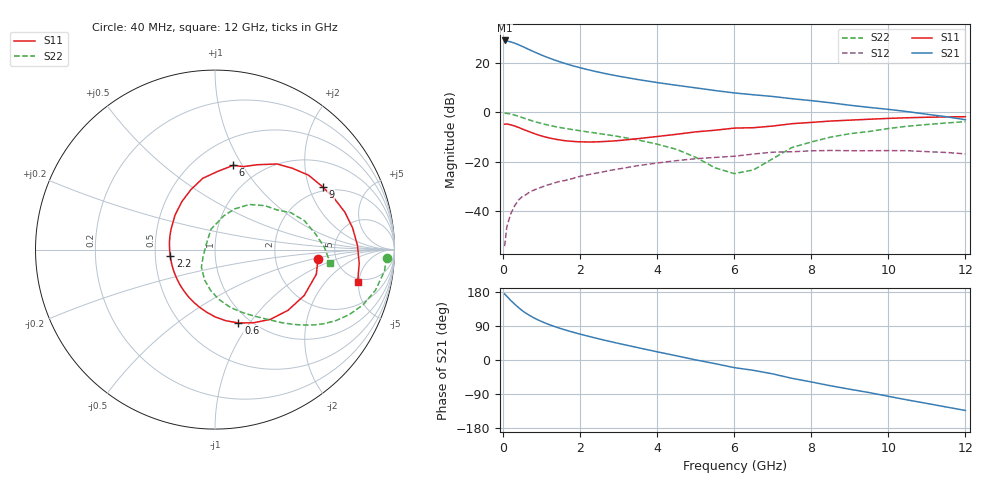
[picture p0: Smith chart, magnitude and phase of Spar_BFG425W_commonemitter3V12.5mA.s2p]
! Filename: 312bfg425.001
! BFG425W Field C1
! V1=8.437E-001V,V2=3.000E+000V, I1=1.606E-004A, I2=1.251E-002A
# GHz  S  MA  R 50
!  S11  S21  S12  S22
!Freq(GHz)  Mag  Ang  Mag  Ang  Mag  Ang  Mag  Ang
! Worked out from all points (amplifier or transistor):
!   44 points, 40 MHz to 12 GHz, reference 50 ohm
!   highest |S21| = 29.0 dB at 40 MHz (marker M1)
!   |S21| within 3 dB of that: start of sweep to 582.3 MHz
!   unconditionally stable (mu >= 1): 1.676 GHz to end of sweep
!   at 700 MHz: K = 0.60, MSG = 28.6 dB, |S12| = -32.0 dB
!   at 2.4 GHz: K = 1.12, MAG = 18.4 dB, |S12| = -24.6 dB
!   at 12 GHz: K = 1.37, MAG = 3.2 dB, |S12| = -16.8 dB
!   S11 on the Smith chart (normalised r, x): 40 MHz: 3.62, -0.58; 600 MHz: 0.88, -0.88; 2.2 GHz: 0.60, -0.05; 6 GHz: 0.75, +0.91; 9 GHz: 1.83, +2.47; 12 GHz: 4.56, -4.84
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0.04  0.576 -5.4  28.06 174.3  0.002 65.3  0.957 -2.7
0.1  0.581 -13.7  27.34 167.9  0.005 81.2  0.952 -7.2
0.2  0.559 -27.2  26.25 157.1  0.009 75.6  0.922 -14.3
0.3  0.529 -39.8  24.71 147.4  0.013 71.4  0.88 -20.5
0.4  0.496 -51.6  23.02 138.4  0.017 66.5  0.831 -25.8
0.5  0.46 -62.5  21.29 130.1  0.02 63.2  0.782 -30.4
0.6  0.429 -72.4  19.57 123.1  0.022 60.8  0.736 -34.1
0.8  0.375 -89.9  16.61 111.3  0.027 56.9  0.656 -39.9
0.9  0.352 -97.5  15.37 106.2  0.029 55.5  0.623 -42.2
1  0.333 -104.8  14.24 101.6  0.031 54.4  0.594 -44.3
1.2  0.304 -118.2  12.37 93.3  0.035 52.6  0.546 -48.0
1.6  0.268 -141.9  9.689 79.7  0.042 50.0  0.475 -54.2
2.2  0.252 -171.5  7.229 63.0  0.055 45.4  0.402 -63.3
3  0.269 156.1  5.344 43.7  0.072 37.5  0.324 -76.6
3.5  0.294 139.3  4.572 32.5  0.084 31.5  0.277 -85.8
4.5  0.36 111.9  3.504 11.1  0.106 17.7  0.179 -108.9
6  0.48 77.9  2.456 -20.1  0.13 -6.0  0.058 144.2
6.5  0.489 71.0  2.254 -27.3  0.144 -8.9  0.069 125.7
8.5  0.666 38.5  1.555 -68.0  0.17 -45.7  0.316 52.7
9  0.694 30.3  1.388 -77.2  0.168 -54.0  0.37 41.5
10.5  0.776 9.0  1.031 -105.5  0.168 -81.1  0.524 17.8
12  0.815 -12.6  0.708 -133.1  0.145 -111.4  0.648 -6.8
